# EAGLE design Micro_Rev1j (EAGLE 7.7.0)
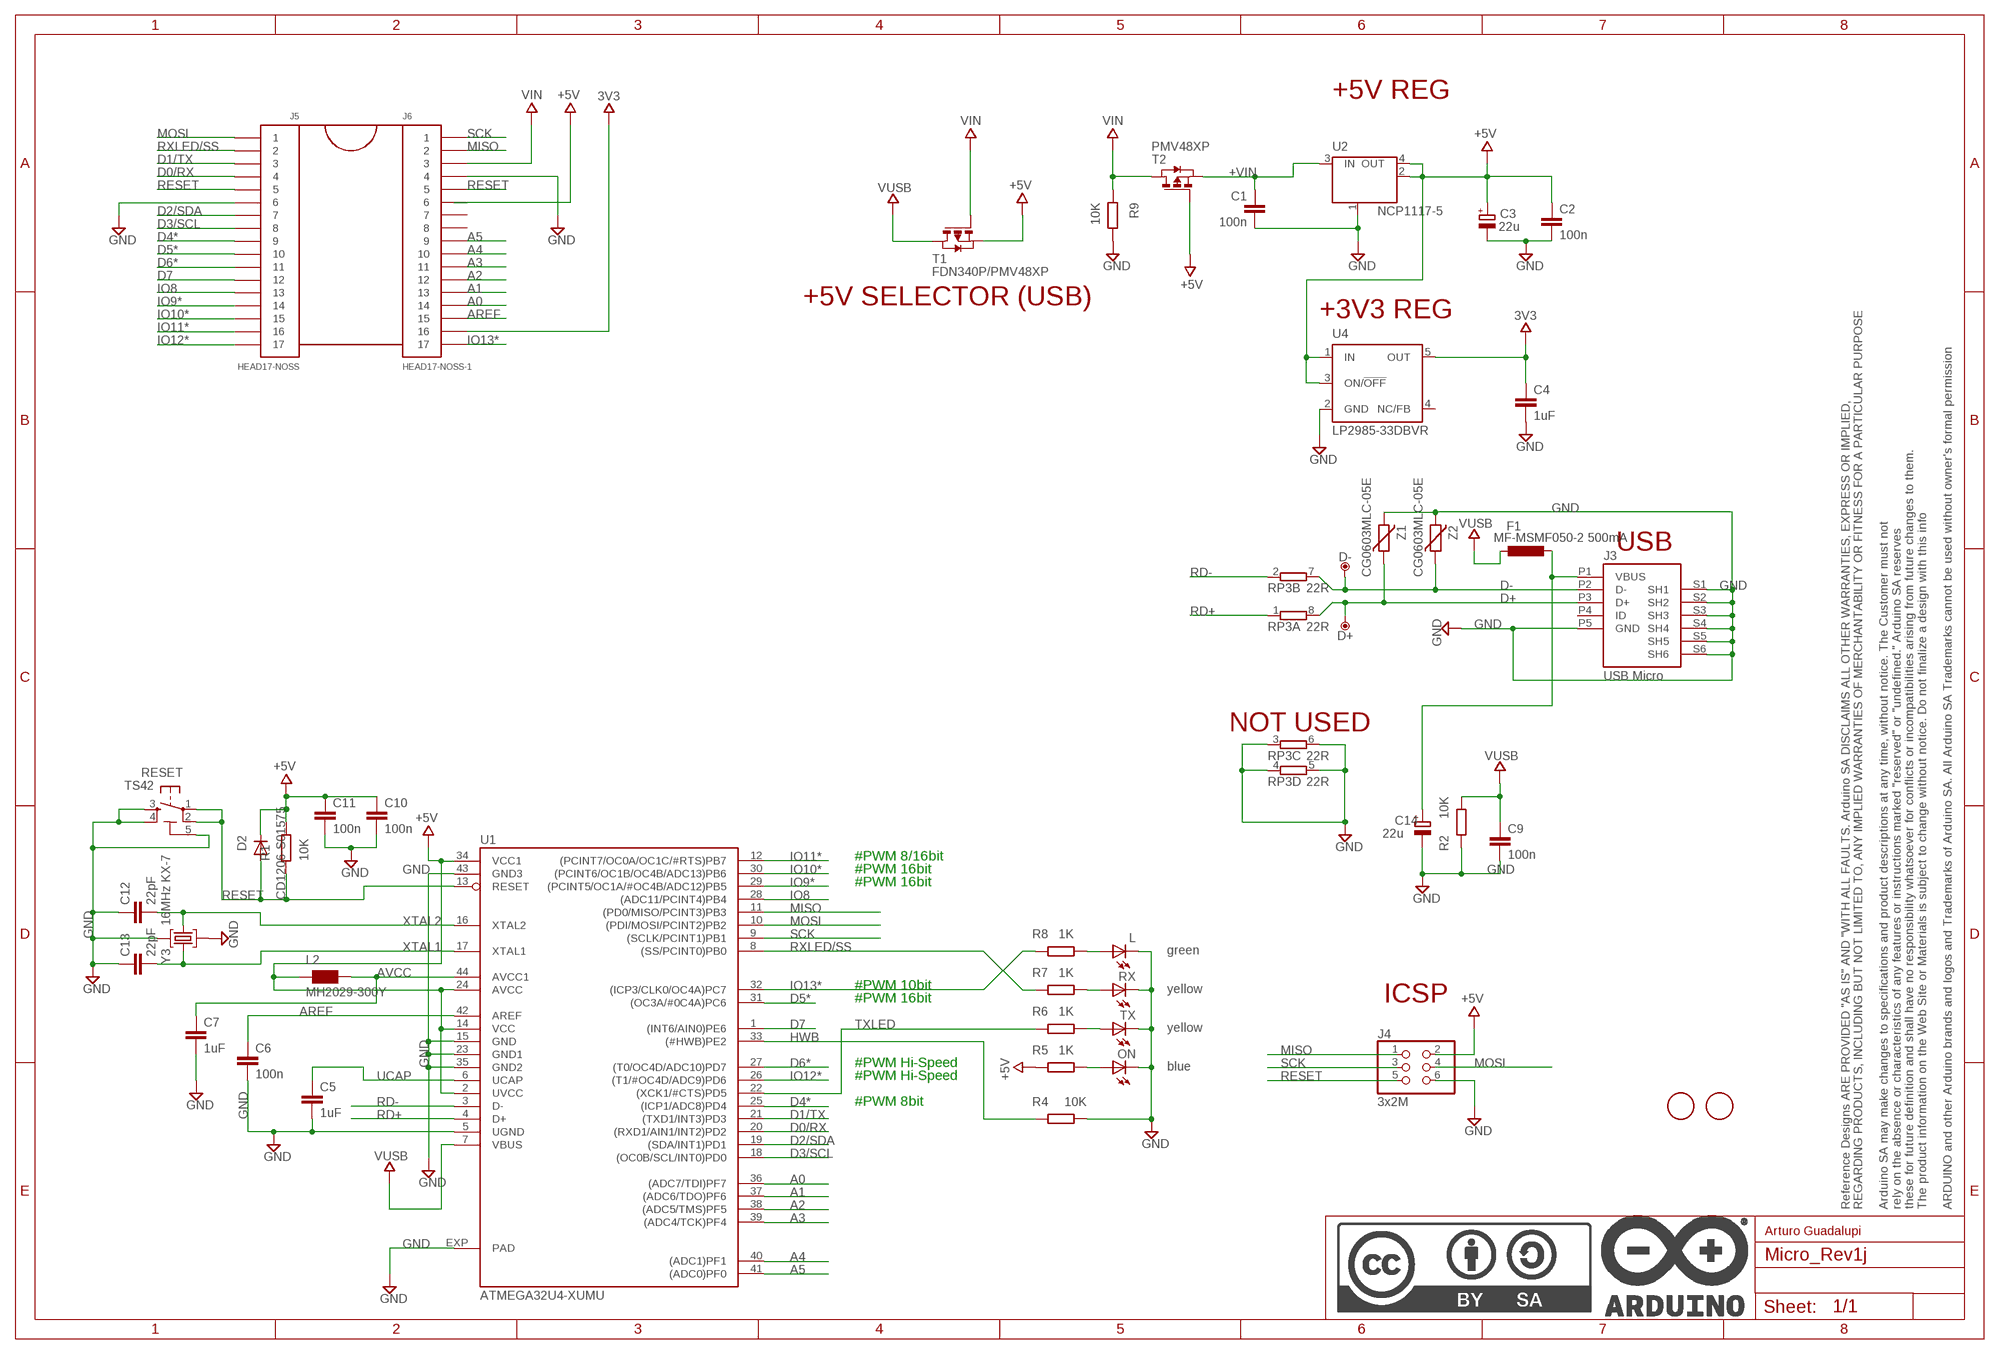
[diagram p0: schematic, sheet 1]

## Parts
C1  100n  C-EUC0402  [C0402]
C2  100n  C-EUC0402  [C0402]
C3  22u  CPOL-EUSMCB  [SMC_B]
C4  1uF  C-EUC0402  [C0402]
C5  1uF  C-EUC0402  [C0402]
C6  100n  C-EUC0402  [C0402]
C7  1uF  C-EUC0402  [C0402]
C9  100n  C-EUC0402  [C0402]
C10  100n  C-EUC0402  [C0402]
C11  100n  C-EUC0402  [C0402]
C12  22pF  C-EUC0402  [C0402]
C13  22pF  C-EUC0402  [C0402]
C14  22u  CPOL-EUSMCB  [SMC_B]
D2  CD1206-S01575  DIODE-MINIMELF  [MINIMELF]
D+  DNP  TPTP-1.00MM  [TP-1.00MM]
D-  DNP  TPTP-1.00MM  [TP-1.00MM]
F1  MF-MSMF050-2 500mA  L-EUL1812  [L1812]
FRAME1  DNP  A3-FRAME  [FRAME]
J3  USB Micro  USB-MICRO-LEGACY  [CON2_USB_MICRO_B_AT]
J4  3x2M  PINHD-2X3  [2X03]
J5  HEAD17-NOSS  [HEAD17-NOSS]
J6  HEAD17-NOSS-1  [HEAD17-NOSS-1]
L  green  LEDCHIPLED_0805  [CHIPLED_0805]
L2  MH2029-300Y  WE-CBF_0805  [0805]
ON  blue  LEDCHIPLED_0805  [CHIPLED_0805]
R1  10K  R-EU_R0402  [R0402]
R2  10K  R-EU_R0402  [R0402]
R4  10K  R-EU_R0402  [R0402]
R5  1K  R-EU_R0402  [R0402]
R6  1K  R-EU_R0402  [R0402]
R7  1K  R-EU_R0402  [R0402]
R8  1K  R-EU_R0402  [R0402]
R9  10K  R-EU_R0402  [R0402]
RESET  TS42  [TS42]
RP3  22R  4R-NCAY16  [CAY16]
RX  yellow  LEDCHIPLED_0805  [CHIPLED_0805]
T1  FDN340P/PMV48XP  PMOSSOT23  [SOT-23]
T2  PMV48XP  PMOSSOT23  [SOT-23]
TX  yellow  LEDCHIPLED_0805  [CHIPLED_0805]
U1  ATMEGA32U4-XUMU  [QFN44ML7X7]
U2  NCP1117-5  LINEAR_MC33269ST  [SOT223]
U4  LP2985-33DBVR  LP2985-XXDBVR33  [SOT23-DBV]
U$37  DNP  FIDUCIAL-1.5MM  [FD-1-1.5]
U$53  DNP  FIDUCIAL-1.5MM  [FD-1-1.5]
Y3  16MHz KX-7  CRYSTAL-3.2-2.5  [CRYSTAL-3.2-2.5]
Z1  CG0603MLC-05E  VARISTORCN0603  [CT/CN0603]
Z2  CG0603MLC-05E  VARISTORCN0603  [CT/CN0603]

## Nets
3V3: C4.1 J6.16 U4.5(OUT)
+5V: C2.1 C3.+ C10.1 C11.1 D2.C J4.2 J6.6 L2.1 R1.1 R5.1 T1.2(S) T2.3(G) U1.2(UVCC) U1.14(VCC) U1.24(AVCC) U1.34(VCC1) U2.2(OUT) U2.4(OUT) U4.1(IN) U4.3(ON/!OFF)
+VIN: C1.1 T2.2(S) U2.3(IN)
A0: J6.14 U1.36((ADC7/TDI)PF7)
A1: J6.13 U1.37((ADC6/TDO)PF6)
A2: J6.12 U1.38((ADC5/TMS)PF5)
A3: J6.11 U1.39((ADC4/TCK)PF4)
A4: J6.10 U1.40((ADC1)PF1)
A5: J6.9 U1.41((ADC0)PF0)
AREF: C6.1 J6.15 U1.42(AREF)
AVCC: C7.1 L2.2 U1.44(AVCC1)
D0/RX: J5.4 U1.20((RXD1/AIN1/INT2)PD2)
D1/TX: J5.3 U1.21((TXD1/INT3)PD3)
D2/SDA: J5.7 U1.19((SDA/INT1)PD1)
D3/SCL: J5.8 U1.18((OC0B/SCL/INT0)PD0)
D4*: J5.9 U1.25((ICP1/ADC8)PD4)
D5*: J5.10 U1.31((OC3A/#0C4A)PC6)
D6*: J5.11 U1.27((T0/OC4D/ADC10)PD7)
D7: J5.12 U1.1((INT6/AIN0)PE6)
D+: D+.X J3.P3(D+) RP3.8 Z1.1
D-: D-.X J3.P2(D-) RP3.7 Z2.1
GND: C1.2 C2.2 C3.- C4.2 C5.2 C6.2 C7.2 C9.2 C10.2 C11.2 C12.1 C13.1 C14.- J3.P5(GND) J3.S1(SH1) J3.S2(SH2) J3.S3(SH3) J3.S4(SH4) J3.S5(SH5) J3.S6(SH6) J4.6 J5.6 J6.4 L.C ON.C R2.1 R4.2 R9.1 RESET.3 RESET.4 RESET.5(5-GND) RP3.3 RP3.4 RP3.5 RP3.6 RX.C TX.C U1.5(UGND) U1.15(GND) U1.23(GND1) U1.35(GND2) U1.43(GND3) U1.EXP(PAD) U2.1(GND/ADJ) U4.2(GND) Y3.2(GND) Y3.4(GND) Z1.2 Z2.2
HWB: R4.1 U1.33((#HWB)PE2)
IO8: J5.13 U1.28((ADC11/PCINT4)PB4)
IO9*: J5.14 U1.29((PCINT5/OC1A/#OC4B/ADC12)PB5)
IO10*: J5.15 U1.30((PCINT6/OC1B/OC4B/ADC13)PB6)
IO11*: J5.16 U1.12((PCINT7/OC0A/OC1C/#RTS)PB7)
IO12*: J5.17 U1.26((T1/#OC4D/ADC9)PD6)
IO13*: J6.17 R8.1 U1.32((ICP3/CLK0/OC4A)PC7)
MISO: J4.1 J6.2 U1.11((PD0/MISO/PCINT3)PB3)
MOSI: J4.4 J5.1 U1.10((PDI/MOSI/PCINT2)PB2)
N$2: R7.2 RX.A
N$3: ON.A R5.2
N$4: R6.2 TX.A
N$7: L.A R8.2
RD+: RP3.1 U1.4(D+)
RD-: RP3.2 U1.3(D-)
RESET: D2.A J4.5 J5.5 J6.5 R1.2 RESET.1 RESET.2 U1.13(RESET)
RXLED/SS: J5.2 R7.1 U1.8((SS/PCINT0)PB0)
SCK: J4.3 J6.1 U1.9((SCLK/PCINT1)PB1)
TXLED: R6.1 U1.22((XCK1/#CTS)PD5)
UCAP: C5.1 U1.6(UCAP)
VIN: J6.3 R9.2 T1.3(G) T2.1(D)
VUSB: C9.1 F1.2 R2.2 T1.1(D) U1.7(VBUS)
VUSBD: C14.+ F1.1 J3.P1(VBUS)
XTAL1: C13.2 U1.17(XTAL1) Y3.3(C2)
XTAL2: C12.2 U1.16(XTAL2) Y3.1(C1)
Unconnected: J3.P4(ID) J6.7 J6.8 U4.4(NC/FB)

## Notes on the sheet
- +5V REG
- +5V SELECTOR (USB)
- +3V3 REG
- USB
- NOT USED
- #PWM 8/16bit
- #PWM 16bit
- #PWM 16bit
- #PWM 10bit
- #PWM 16bit | ICSP
- #PWM Hi-Speed
- #PWM Hi-Speed
- #PWM 8bit
- Arturo Guadalupi

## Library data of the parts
C1 C2 C4-C7 C9-C13 = gen_comp:C-EU: CAPACITOR, European symbol
C3 C14 = rcl:CPOL-EU: POLARIZED CAPACITOR, European symbol
D2 = diode:DIODE-: DIODE
D+ D- = Arduino-utility:TP: Testpoint; DATASHEET: DNP; DISTRIBUTOR-LINK: DNP; DISTRIBUTOR-PN: DNP; MANUFACTURER: DNP; MANUFACTURER-PN: DNP
F1 = rcl:L-EU: INDUCTOR, European symbol
FRAME1 = Arduino-utility:A3-FRAME; CODE-ARDUINO: DNP; DATASHEET: DNP; DISTRIBUTOR-LINK: DNP; DISTRIBUTOR-PN: DNP; MANUFACTURER: DNP; MANUFACTURER-PN: DNP; NOTE: DNP
J3 = Arduino-connectors:USB-MICRO-LEGACY; DATASHEET: http://media.digikey.com/pdf/Data%20Sheets/FCI%20PDFs/10118193-0001LF_Webpage.PDF; DISTRIBUTOR-LINK: http://www.digikey.it/product-detail/en/10118193-0001LF/609-4616-2-ND/2785388; DISTRIBUTOR-PN: 609-4616-2-ND; MANUFACTURER: FCI; MANUFACTURER-PN: 10118193-0001LF
J4 = gen_comp:PINHD-2X3: PIN HEADER
J5 = gen_comp:HEAD17-NOSS
J6 = gen_comp:HEAD17-NOSS-1
L ON RX TX = led:LED: LED
L2 = wuerth-elektronik:WE-CBF: SMD EMI Suppression Ferrite Beads
R1 R2 R4-R9 = gen_comp:R-EU_: RESISTOR, European symbol
RESET = Arduino:TS42: TS42 Dongnan Electronics Tact switch VDC 12V - 50mA
RP3 = resistor-dil:4R-N: Array Chip Resistor Source: RS Component / Phycomp
T1 T2 = zetex:PMOSSOT23: MOS FET
U1 = gen_comp:ATMEGA32U4-XU
U2 = gen_comp:LINEAR_MC33269ST*: Adjustable Output Low Dropout Voltage Regulator 800 mA Source: http://www.onsemi.com/pub/Collateral/MC33269-D.PDF
U4 = gen_comp:LP2985-XXDBVR: ULTRALOW-POWER 50-mA LOW-DROPOUT LINEAR REGULATORS 50-mA Low-Dropout Regulator Source: http://focus.ti.com/lit/ds/symlink/tps77001.pdf
U$37 U$53 = Arduino-utility:FIDUCIAL: Fiducial mount; DATASHEET: DNP; DISTRIBUTOR-LINK: DNP; DISTRIBUTOR-PN: DNP; MANUFACTURER: DNP; MANUFACTURER-PN: DNP
Y3 = gen_comp:CRYSTAL-3.2-2.5
Z1 Z2 = varistor:VARISTOR: VARISTOR

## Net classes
0 default: width 0.254 mm, drill 0.5 mm, clearance 0.203 mm

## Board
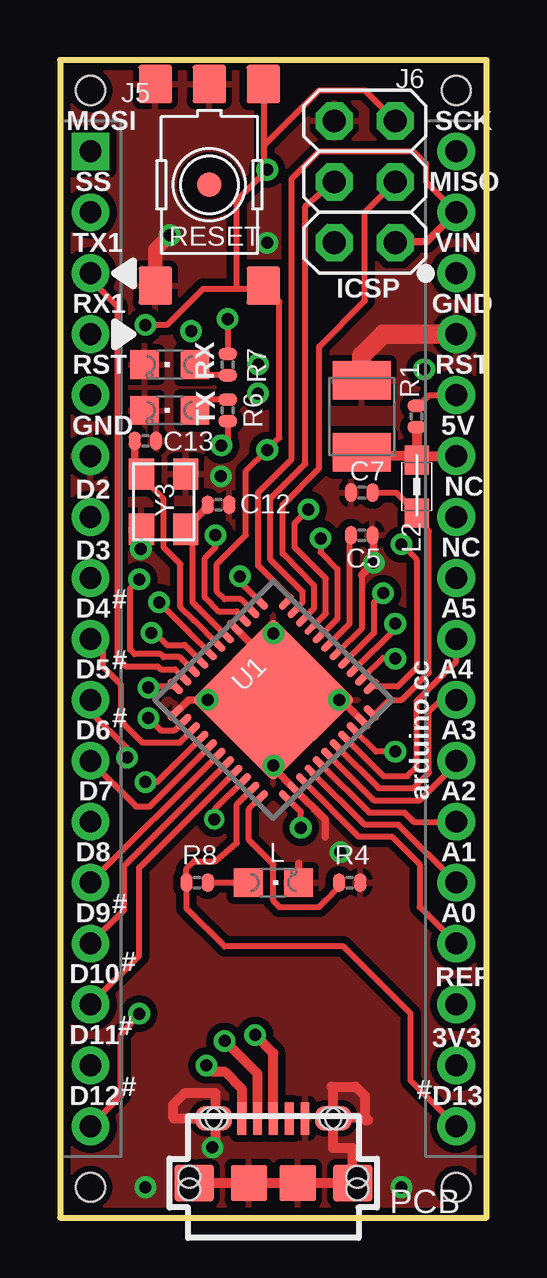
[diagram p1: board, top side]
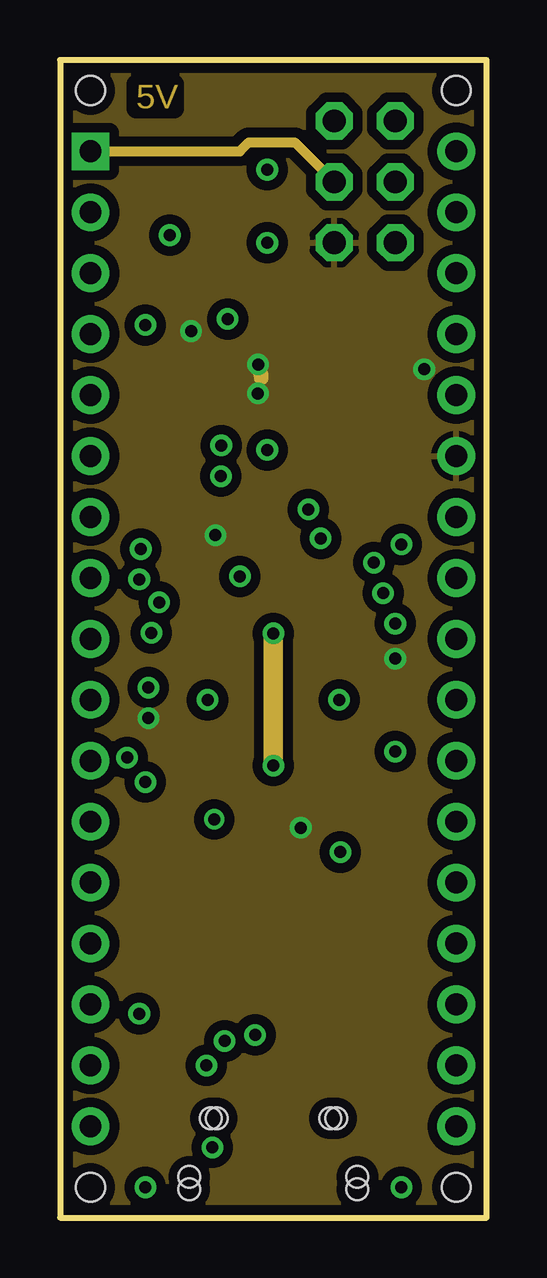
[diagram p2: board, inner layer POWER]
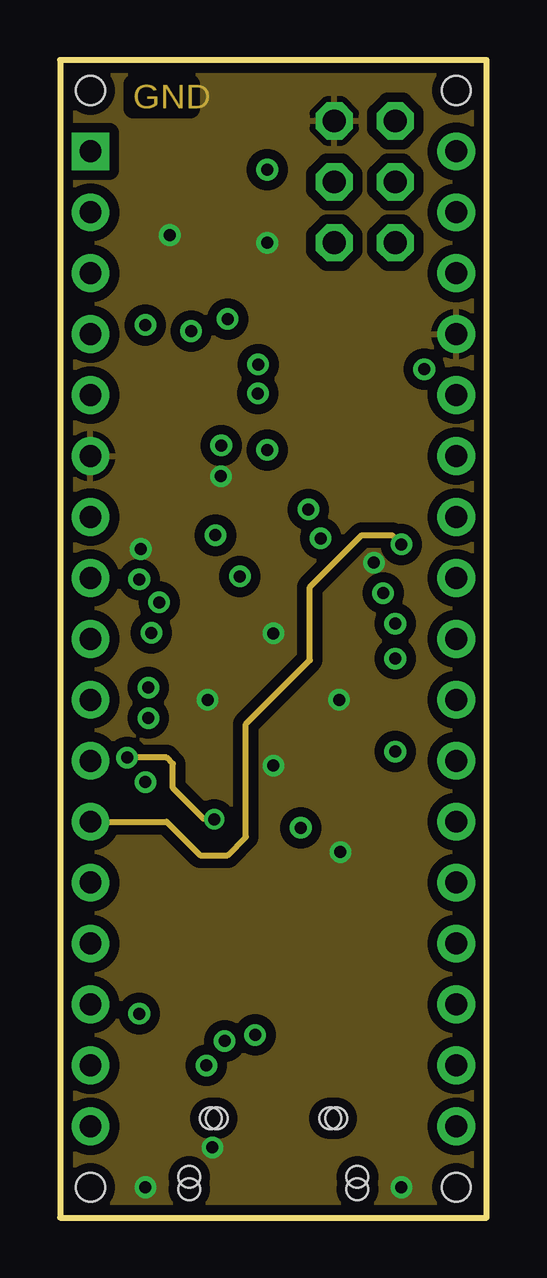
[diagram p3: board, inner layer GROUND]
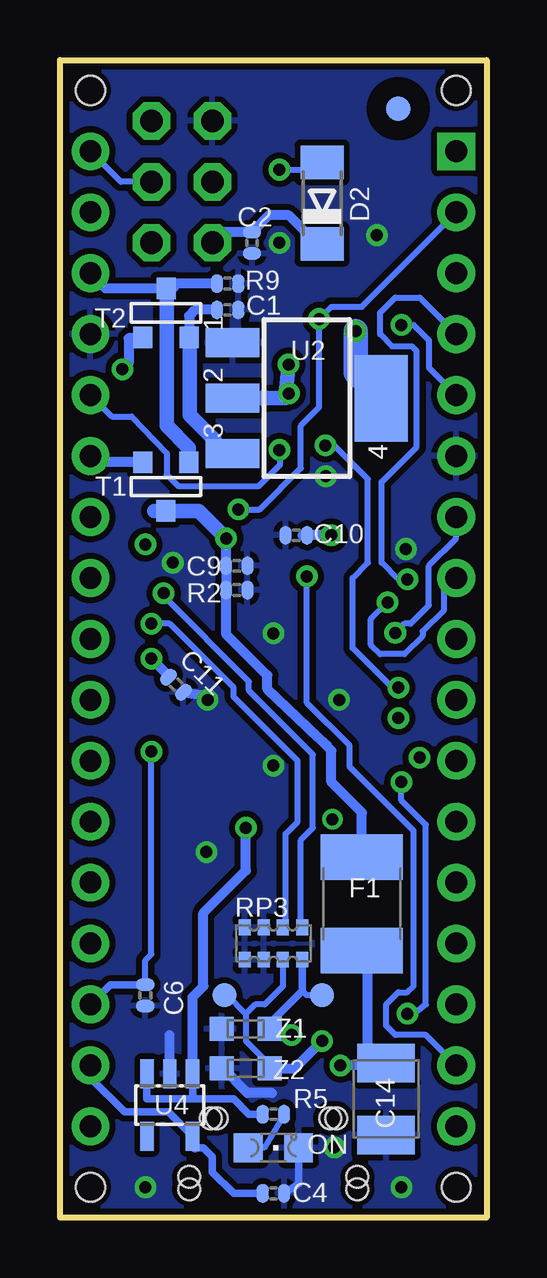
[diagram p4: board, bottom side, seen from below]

Size 17.78 x 48.26 mm. Coordinates in mm from the lower left corner, seen from the top.
Outline: 0,0 17.78,0 17.78,48.26 0,48.26 0,0
Copper layers (1*2*15*16): Top 0.035mm / dielectric 0.2mm / POWER 0.0175mm / dielectric 0.3mm / GROUND 0.0175mm / dielectric 0.2mm / Bottom 0.035mm
Design rules "SystemElettronica": minimum track width 6mil, minimum drill 0.499mm, track to track 6mil, track to pad 6mil, pad to pad 5mil, via to via 5mil, smd to smd 0mil, copper to edge 10mil, drill to drill 8mil, minimum pad ring 6mil, minimum via ring 4mil, stop-mask expansion 4mil, vias tented up to drill 25mil, thermal gap 10mil
Holes 1.2 mm at 1.27,1.27 16.51,1.27 1.27,46.99 16.51,46.99

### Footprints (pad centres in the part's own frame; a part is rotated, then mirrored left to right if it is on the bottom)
C0402 = smd 0.508 x 0.762: 1 -0.445,0; 2 0.445,0
SMC_B = smd 1.6 x 2.4: + -1.5,0; - 1.5,0
MINIMELF = smd 1.4 x 1.8: A 1.7,0; C -1.7,0
TP-1.00MM = smd 1 x 1 bottom: X 0,0
L1812 = smd 1.9 x 3.4: 1 -1.95,0; 2 1.95,0
CON2_USB_MICRO_B_AT = smd 0.406 x 1.346: P1 -1.321,2.692; P2 -0.66,2.692; P3 0,2.692; P4 0.66,2.692; P5 1.321,2.692 | smd 1.651 x 1.549: S1 -3.302,0; S2 3.302,0 | smd 1.524 x 1.016: S3 -2.489,2.692; S4 2.489,2.692 | smd 1.524 x 1.524: S5 -1.016,0; S6 1.016,0 | hole 0.9: -3.505,0.254; -3.505,-0.254; 3.505,0.254; 3.505,-0.254; -2.616,2.692; -2.362,2.692; 2.362,2.692; 2.616,2.692
2X03 = drill 0.95 pad 1.55 octagon: 1 -2.54,-1.27; 2 -2.54,1.27; 3 0,-1.27; 4 0,1.27; 5 2.54,-1.27; 6 2.54,1.27
HEAD17-NOSS = drill 0.914 pad 1.575 square: 1 0,0 | drill 0.914 pad 1.575: 2 2.54,0; 3 5.08,0; 4 7.62,0; 5 10.16,0; 6 12.7,0; 7 15.24,0; 8 17.78,0; 9 20.32,0; 10 22.86,0; 11 25.4,0; 12 27.94,0; 13 30.48,0; 14 33.02,0; 15 35.56,0; 16 38.1,0; 17 40.64,0
HEAD17-NOSS-1 = drill 0.914 pad 1.575: 1 0,0; 2 2.54,0; 3 5.08,0; 4 7.62,0; 5 10.16,0; 6 12.7,0; 7 15.24,0; 8 17.78,0; 9 20.32,0; 10 22.86,0; 11 25.4,0; 12 27.94,0; 13 30.48,0; 14 33.02,0; 15 35.56,0; 16 38.1,0; 17 40.64,0
CHIPLED_0805 = smd 1.2 x 1.2: A 0,-1.05; C 0,1.05
0805 = smd 1.2 x 1: 1 -1.1,0; 2 1.1,0
R0402 = smd 0.508 x 0.762: 1 -0.445,0; 2 0.445,0
TS42 = smd 1.6 x 1.4: 1 -4.2,2.25; 2 4.2,2.25; 3 -4.2,-2.25; 4 4.2,-2.25; 5 -4.2,0
CAY16 = smd 0.5 x 0.65: 1 -1.2,-0.675; 2 -0.4,-0.675; 3 0.4,-0.675; 4 1.2,-0.675; 5 1.2,0.675; 6 0.4,0.675; 7 -0.4,0.675; 8 -1.2,0.675
SOT-23 = smd 0.787 x 0.889: 1 0.025,-1.016; 2 -0.94,1.016; 3 0.991,1.016
QFN44ML7X7 = smd 0.75 x 0.275: 1 -3.275,2.5; 2 -3.275,2; 3 -3.275,1.5; 4 -3.275,1; 5 -3.275,0.5; 6 -3.275,0; 7 -3.275,-0.5; 8 -3.275,-1; 9 -3.275,-1.5; 10 -3.275,-2; 11 -3.275,-2.5; 23 3.275,-2.5; 24 3.275,-2; 25 3.275,-1.5; 26 3.275,-1; 27 3.275,-0.5; 28 3.275,0; 29 3.275,0.5; 30 3.275,1; 31 3.275,1.5; 32 3.275,2; 33 3.275,2.5 | smd 0.275 x 0.75: 12 -2.5,-3.275; 13 -2,-3.275; 14 -1.5,-3.275; 15 -1,-3.275; 16 -0.5,-3.275; 17 0,-3.275; 18 0.5,-3.275; 19 1,-3.275; 20 1.5,-3.275; 21 2,-3.275; 22 2.5,-3.275; 34 2.5,3.275; 35 2,3.275; 36 1.5,3.275; 37 1,3.275; 38 0.5,3.275; 39 0,3.275; 40 -0.5,3.275; 41 -1,3.275; 42 -1.5,3.275; 43 -2,3.275; 44 -2.5,3.275 | smd 4.826 x 4.826: EXP 0,0
SOT223 = smd 1.219 x 2.235: 1 -2.311,-3.099; 2 0,-3.099; 3 2.311,-3.099 | smd 3.6 x 2.2: 4 0,3.099
SOT23-DBV = smd 0.55 x 1.2: 1 -0.95,-1.3; 2 0,-1.3; 3 0.95,-1.3; 4 0.95,1.3; 5 -0.95,1.3
FD-1-1.5 = smd 1.016 x 1.016: P$1 0,0
CRYSTAL-3.2-2.5 = smd 1.3 x 1.05: 1 -1.15,-0.925; 2 1.15,-0.925; 3 1.15,0.925; 4 -1.15,0.925
CT/CN0603 = smd 1 x 1: 1 -1,0; 2 1,0

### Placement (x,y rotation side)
C1  10.79,37.85 0 bottom
C2  9.78,40.64 270 bottom
C3  12.57,33.4 90 top
C4  8.89,1.02 0 bottom
C5  12.57,28.45 0 top
C6  14.22,9.27 270 bottom
C7  12.57,30.23 180 top
C9  10.41,27.18 0 bottom
C10  7.94,28.45 180 bottom
C11  12.95,22.23 315 bottom
C12  6.6,29.72 180 top
C13  3.56,32.38 180 top
C14  4.19,4.95 270 bottom
D2  6.86,42.29 90 bottom
D+  6.86,9.27 0 top
D-  10.92,9.27 0 top
F1  5.21,13.08 90 bottom
FRAME1  0,0 0 top
J3  8.89,1.45 0 top
J4  12.7,43.18 90 top
J5  1.27,44.45 270 top
J6  16.51,44.45 270 top
L  8.89,13.97 270 top
L2  14.86,30.48 270 top
ON  8.89,2.92 270 bottom
R1  14.86,33.4 90 top
R2  10.41,26.16 180 bottom
R4  12.06,13.97 0 top
R5  8.89,4.32 0 bottom
R6  6.99,33.66 90 top
R7  6.99,35.56 270 top
R8  5.71,13.97 0 top
R9  10.79,38.94 180 bottom
RESET  6.22,43.05 270 top
RP3  8.89,11.43 180 bottom
RX  4.57,35.56 90 top
T1  13.4,30.48 0 bottom
T2  13.34,37.72 180 bottom
TX  4.57,33.66 90 top
U1  8.89,21.59 225 top
U2  7.49,34.16 270 bottom
U4  13.21,4.7 180 bottom
U$37  6.22,43.05 0 top
U$53  3.68,46.23 0 bottom
Y3  4.32,29.84 90 top
Z1  10.03,7.87 180 bottom
Z2  10.03,6.22 180 bottom

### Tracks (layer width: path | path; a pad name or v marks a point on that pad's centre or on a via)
3V3
  Bottom 0.305: U4.5 13.28,4.42 15.09,4.42 16.51,5.84 J6.16 | 12.16,2.92 11.81,2.92 11.43,2.54 11.43,1.91 10.54,1.02 C4.1
  Bottom 0.406: 12.16,2.92 U4.5
+5V  (via drill 0.5 pad 0.9)
  Top 0.254: U1.24 4.79,20.32 4.19,20.32 v3.68,20.83 | U1.14 7.37,25.27 6.6,25.27 6.03,25.84 6.03,27.5 6.48,27.94 v6.48,28.45 | U1.2 13.46,23.33 v13.97,23.3 | U1.34 10.03,16.91 v10.03,16.26
  Top 0.406: R1.1 L2.1 14.73,31.58 14.73,31.75 | 14.73,31.75 J6.6 | 14.73,31.75 12.57,31.75 C3.+
  POWER 0.61: v8.26,35.57 8.38,35.06 8.38,35.14 8.39,35.14 8.39,35
  Bottom 0.305: U4.1 12.26,4.95 | 12.26,4.95 10.54,4.95 9.91,4.32 R5.1 | U4.3 14.16,4.95 12.26,4.95
  Bottom 0.406: v10.03,16.26 10.03,14.48 11.81,12.7 11.81,9.65 12.26,9.21 U4.1 | C11.1 13.41,22.75 v13.97,23.3 | 7.68,28.45 C10.1 v6.48,28.45 | D2.C 7.06,40.59 8.26,41.78 9.08,41.78 C2.1 10.99,41.08 J4.2 | T1.2 16.26,31.5 J6.6 | T2.3 14.92,36.66 14.92,35.62 v15.18,35.37
  Bottom 0.61: U2.2 8.38,34.16 v8.26,35.57
  Bottom 1.016: v5.46,36.96 5.46,35.23 U2.4
  other vias: 8.25,34.36
  pour POWER (isolate 0.406): -0.64,48.9 18.41,48.9 18.41,-0.64 -0.64,-0.64
+VIN
  Bottom 0.406: C1.1 12.14,37.85 12.39,37.59 T2.2
  Bottom 0.61: U2.3 11.34,31.85 11.34,32.42 12.38,33.47 12.38,35.99 T2.2
A0
  Top 0.254: U1.36 12.45,15.88 13.84,15.88 14.99,14.73 14.99,12.95 J6.14
A1
  Top 0.254: U1.37 12.7,16.38 14.1,16.38 J6.13
A2
  Top 0.254: U1.38 12.88,16.89 | 12.88,16.89 | 12.88,16.89 14.35,16.89 14.73,16.51 J6.12
A3
  Top 0.254: U1.39 13.08,17.4 14.99,17.4 16.26,18.67 J6.11
A4
  Top 0.254: U1.40 13.28,17.91 14.73,17.91 15.37,18.54 15.37,21.08 15.88,21.59 J6.10
A5
  Top 0.254: U1.41 13.48,18.41 14.48,18.41 14.86,18.8 14.86,21.54 16.51,23.19 J6.9
AREF  (via drill 0.5 pad 0.9)
  Top 0.254: U1.42 13.17,19.43 v13.97,19.43
  Bottom 0.254: v13.97,19.43 13.97,10.99 14.22,10.73 C6.1
  Bottom 0.305: C6.1 15.68,9.72 J6.15
AVCC
  Top 0.254: U1.44 13.17,21.04 13.72,21.59 14.24,21.59 15.37,22.72 15.37,28.62 L2.2 14.01,30.23 C7.1
D0/RX  (via drill 0.5 pad 0.9)
  Top 0.254: U1.20 4.99,23.37 4.32,23.37 4.19,23.5 3.11,23.5 2.92,23.69 2.92,26.23 v3.3,26.61
  Bottom 0.254: v3.3,26.61 3.68,26.61 4.38,27.3 4.38,30.67 2.92,32.13 2.92,36.13 3.11,36.32 3.94,36.32 4.45,36.83 4.45,37.72 3.81,38.35 2.79,38.35 J5.4
D1/TX
  Top 0.254: U1.21 4.79,22.86 4.19,22.86 4.06,22.99 2.73,22.99 2.41,23.3 2.41,37.97 1.27,39.12 J5.3
D2/SDA  (via drill 0.5 pad 0.9)
  Top 0.254: U1.19 5.19,23.88 4.45,23.88 3.94,24.38 v3.81,24.38
  Bottom 0.254: v3.81,24.38 3.43,24.77 3.17,24.77 2.41,25.53 2.41,27.18 1.27,28.32 J5.7
D3/SCL  (via drill 0.5 pad 0.9)
  Top 0.254: U1.18 5.39,24.38 5.4,24.38 v4.13,25.65
  Bottom 0.254: v4.13,25.65 4.83,24.96 4.83,23.88 4.45,23.5 3.43,23.5 2.67,24.26 2.67,24.45 1.78,25.34 1.78,26.16 J5.8
D4*
  Top 0.254: U1.25 4.99,19.81 3.43,19.81 2.54,20.7 2.54,22.23 1.78,22.99 1.78,23.62 J5.9
D5*  (via drill 0.5 pad 0.85, 0.5 pad 0.9)
  Top 0.254: U1.31 6.48,17.06 v6.43,16.61 | J5.10 1.27,21.08 2.79,19.56 v2.79,19.18
  GROUND 0.254: v2.79,19.18 4.45,19.18 4.7,18.92 4.7,17.91 5.97,16.64 v6.43,16.61
D6*
  Top 0.254: U1.27 3.74,17.14 3.17,17.14 J5.11
D7  (via drill 0.5 pad 0.9)
  Top 0.254: U1.1 14.06,22.14 14.06,22.13 14.86,22.94 14.86,27.43 v14.22,28.07
  GROUND 0.254: J5.12 4.45,16.51 5.84,15.11 6.99,15.11 7.75,15.88 7.75,20.57 10.41,23.24 10.41,26.29 12.57,28.45 13.84,28.45 v14.22,28.07
D+  (via drill 0.5 pad 0.9)
  Top 0.406: J3.P3 8.89,6.86 v8.13,7.62
  Bottom 0.254: D+.X 7.51,9.27 7.69,9.46
  Bottom 0.305: RP3.8 7.69,9.46 9.27,7.87 9.14,7.87
  Bottom 0.406: v8.13,7.62 Z1.1 9.14,7.87
D-  (via drill 0.5 pad 0.9)
  Top 0.406: J3.P2 8.23,5.99 v6.86,7.37
  Bottom 0.254: RP3.7 8.49,9.65 9.25,8.89 9.65,8.89 10.03,8.51 | 10.03,8.51 10.03,7.37 9.03,6.37 Z2.1 | D-.X 10.79,9.27 10.03,8.51
  Bottom 0.406: Z2.1 8,6.22 v6.86,7.37
GND  (via drill 0.5 pad 0.9)
  Top 0.254: U1.EXP v8.89,24.36 | U1.5 12.57,24.57 12.57,26.8 | 13.04,28.19 C5.2
  Top 0.305: U1.EXP 8.89,18.76 U1.35 11.05,16.6 11.05,15.88 | U1.23 5.35,21.59 U1.EXP | U1.15 8.89,23 U1.EXP | L.C 9.94,14.77 | 12.57,26.8 v13.08,27.3 13.08,28.28 13.04,28.19 | U1.43 11.72,21.59 v11.63,21.59
  Top 0.406: J3.S1 J3.S2 12.19,2.9 11.38,2.9 J3.S4 | 6.22,3.05 v6.35,2.93 6.48,3.05 6.48,5.21 5.21,5.21 4.7,4.7 4.7,4.19 4.75,4.14 J3.S3 | J3.S4 11.38,5.38 11.3,5.46 12.32,5.46 12.7,5.08 12.7,4.19 12.83,4.06 12.7,4.06 12.57,4.19 11.43,4.19 J3.S4
  Top 0.61: RESET.4 3.97,40.36 v4.57,40.96 | Y3.4 3.39,28.09 v3.37,27.88
  Top 0.813: C3.- 12.57,35.94 13.46,36.83 J6.4
  POWER 0.813: v8.89,24.36 v8.89,18.85
  Bottom 0.305: ON.C 7.84,1.42 C4.2
  Bottom 0.406: U4.2 13.21,7.62 | C11.2 11.81,21.77 v11.63,21.59 | 8.95,5.21 9.97,5.21 11.05,6.29
  other vias: 11.68,15.24 6.71,30.91 6.15,21.59 3.56,1.27 14.22,1.27 8.64,40.64
  pour GROUND (isolate 0.406): -1.27,49.53 19.05,49.53 19.05,-1.27 -1.27,-1.27
  pour Bottom (isolate 0.254): 19.68,50.16 -1.91,50.16 -1.91,-1.91 19.68,-1.91
  pour Top (isolate 0.305): -2.54,50.8 20.32,50.8 20.32,-2.54 -2.54,-2.54
HWB
  Top 0.254: U1.33 7.87,17.04 7.87,15.75 8.89,14.73 8.89,13.21 9.14,12.95 10.79,12.95 11.05,13.21 11.56,13.73 R4.1
IO8
  Top 0.254: J5.13 U1.28
IO9*
  Top 0.254: U1.29 2.67,14.66 2.67,12.83 J5.14
IO10*
  Top 0.254: U1.30 3.3,14.59 3.3,10.92 J5.15
IO11*  (via drill 0.5 pad 0.9)
  Top 0.254: U1.12 7.49,26.52 v7.49,26.73
  Bottom 0.254: v7.49,26.73 7.49,21.46 5.71,19.68 5.71,18.8 3.05,16.13 3.05,9.65 3.3,9.4 3.68,9.4 4.19,8.89 4.19,8 3.81,7.62 2.54,7.62 J5.16
IO12*  (via drill 0.5 pad 0.9)
  Top 0.254: J5.17 2.54,5.08 2.54,7.62 v3.3,8.51 | U1.26 4.05,18.16 v3.56,18.16
  Bottom 0.254: v3.3,8.51 3.05,8.51 2.54,8.89 2.54,16.38 3.56,17.4 v3.56,18.16
IO13*
  Top 0.254: J6.17 14.61,5.71 14.61,8.51 11.81,11.3 6.86,11.3 5.27,12.89 R8.1 5.27,14.54 5.59,14.86 6.48,14.86 7.37,15.62 7.37,17.24 U1.32
MISO
  Top 0.254: U1.11 9.53,25.76 9.53,25.91 8.26,27.18 8.26,30.23 9.65,31.62 9.65,43.31 10.79,44.45 14.73,44.45 15.24,43.94 15.24,43.18 J6.2
  Top 0.305: J6.2 15.28,40.68 14.01,40.68 J4.1
MOSI
  Top 0.254: U1.10 10.11,25.66 10.11,26.09 8.76,27.43 8.76,29.97 10.22,31.43 10.22,42.16 J4.4
  POWER 0.406: J5.1 7.49,44.45 7.87,44.83 9.78,44.83 J4.4
N$2
  Top 0.254: R7.2 5.91,35.12 5.46,35.56 RX.A 5.59,35.56
N$3
  Bottom 0.254: R5.2 9.27,2.92 ON.A
N$4
  Top 0.254: R6.2 6.07,34.1 TX.A
N$7
  Top 0.254: R8.2 L.A
RD+  (via drill 0.5 pad 0.9)
  Top 0.254: U1.4 13.08,24.37 13.08,25.65 v13.46,26.04
  Bottom 0.254: v13.46,26.04 13.46,25.91 9.91,22.35 9.91,21.97 7.24,19.3 7.24,16.26 7.75,15.75 7.75,11.91 RP3.1
RD-  (via drill 0.5 pad 0.9)
  Top 0.254: U1.3 13.97,24.55 v13.97,24.77
  Bottom 0.254: v13.97,24.77 13.21,24.77 10.54,22.1 10.54,21.72 7.87,19.05 7.87,16.51 8.38,16 8.38,11.96 RP3.2
RESET  (via drill 0.5 pad 0.9)
  Top 0.254: U1.13 7.53,25.78 6.86,25.78 6.54,26.1 6.54,27.24 7.75,28.45 7.75,31.11 v8.64,32 9.14,32.51 9.14,38.18 RESET.2 | v8.64,43.69 8.51,43.69 8.51,43.81 | 8.51,43.81 8.51,44.7 | 8.51,44.7 10.79,46.99 12.7,46.99 J4.5 | v3.56,37.21 4.45,37.21 5.96,38.73 8.51,38.73 8.38,38.85 8.38,38.86 8.51,38.86 | RESET.2 8.64,38.85 8.64,38.73 8.51,38.73 | 8.51,38.82 RESET.2 | 8.22,39.11 RESET.2 | RESET.2 8.45,38.83 8.45,38.92 8.47,38.77 | v8.64,43.69 7.37,42.42 7.37,38.73 8.51,38.73 | 8.51,38.73 8.51,38.86 | 8.51,38.86 8.47,38.9 RESET.2 | 8.47,38.77 RESET.2 | 8.47,38.77 8.51,38.73 | 14.9,33.85 14.95,33.85 15.39,34.29 J6.5 | v8.64,43.69 8.51,43.81 | 8.51,44.7 8.51,47.22 RESET.1
  Top 0.305: 14.9,33.85 R1.2
  Bottom 0.254: J5.5 2.41,35.43 2.41,36.58 3.05,37.21 v3.56,37.21 | J6.5 15.62,33.4 14.8,33.4 13.34,31.88 13.34,30.99 12.83,30.48 9.53,30.48 8.61,31.39 8.61,31.85 v8.64,32 | v8.64,43.69 6.86,43.69 D2.A 6.86,44.07
RXLED/SS  (via drill 0.5 pad 0.9)
  Top 0.254: U1.8 11.07,25.19 11.07,26.64 9.78,27.94 9.78,28.96 v10.35,29.53 | v6.99,37.47 R7.1
  Bottom 0.254: v10.35,29.53 9.46,29.53 7.75,31.24 7.75,33.02 6.99,33.78 v6.99,37.47 6.48,37.97 5.21,37.97 J5.2
SCK
  Top 0.254: U1.9 10.59,25.41 10.59,26.34 9.27,27.69 9.27,29.72 10.79,31.24 10.79,36.32 12.7,38.23 12.7,41.91 J4.3
  Bottom 0.254: J4.3 15.24,43.18 J6.1
TXLED  (via drill 0.5 pad 0.9)
  Top 0.254: U1.22 3.77,22.14 v3.68,22.1 | R6.1 6.99,32.46 v6.72,32.19
  Bottom 0.254: v3.68,22.1 3.94,22.1 5.59,23.75 5.59,26.67 4.95,27.3 4.95,30.79 6.36,32.19 v6.72,32.19
UCAP
  Top 0.254: U1.6 12.06,24.77 12.06,28.45 12.08,28.43 C5.1
VIN
  Bottom 0.406: J6.3 15.88,38.73 T2.1 13.08,38.73 12.9,38.94 R9.2
  Bottom 0.61: T1.3 12.41,32.09 13.34,33.02 13.34,38.2 T2.1
VUSB  (via drill 0.5 pad 0.9)
  Top 0.254: U1.7 11.56,24.96 11.56,27.05 10.86,27.75 v10.86,28.32
  Bottom 0.254: 13.72,29.46 13.84,29.46
  Bottom 0.406: 6.6,19.62 6.83,19.84 7.03,20.03 | 7.03,20.03 9.14,22.04 9.14,22.61 10.83,24.3 10.86,24.36 R2.2 C9.1 v10.86,28.32 10.82,28.42 10.9,28.42 | F1.2 5.21,16.89 6.48,18.16 6.48,19.47 7.03,20.03
  Bottom 0.61: 13.84,29.46 T1.1 | T1.1 13.72,29.46 | T1.1 12,29.46 v10.86,28.32
VUSBD  (via drill 0.5 pad 0.9)
  Top 0.406: J3.P1 7.57,5.38 6.86,6.1 6.35,6.1 v6.1,6.35
  Bottom 0.406: F1.1 4.95,10.62 4.95,7.21 C14.+ 4.09,6.35 v6.1,6.35
XTAL1
  Top 0.254: U1.17 5.59,24.89 5.02,25.46 5.02,27.24 4.32,27.94 4.32,29.97 3.46,30.83 | 3.56,30.83 3.46,30.83 | 3.46,30.83 3.43,30.86
  Top 0.305: C13.2 3.11,30.97 Y3.3 3.56,30.83
XTAL2
  Top 0.254: U1.16 5.79,25.4 5.52,25.65 5.52,25.72 5.52,28.37 5.23,28.68 Y3.1 5.21,28.7
  Top 0.305: C12.2 6.16,29.65 5.59,29.08 5.59,29.04 Y3.1

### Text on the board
POWER: 5V
GROUND: GND
tPlace: MOSI | SCK | SS | MISO | TX1 | VIN | RX1 | ICSP | GND | RST | RX | RST | GND | TX | 5V | D2 | NC | NC | D3 | D4 | # | A5 | # | D5 | A4 | D6 | # | A3 | D7 | A2 | D8 | A1 | # | D9 | A0 | D10 | # | REF | # | D11 | 3V3 | D12 | # | # | D13
tNames: arduino.cc
test-probe: MICRO / TEST POINTS | ISP1_4 | ISP1_3 | SS | ISP1_1 | 0 | DC_VIN+ | 1 | 5V_REF | DC_VIN- | ISP1_5 | USB1_GND | USB1_5V | 2 | 3 | 4 | A5 | 5 | A4 | 6 | A3 | 7 | A2 | 8 | A1 | 9 | A0 | USB_D+ | USB_D- | 10 | AREF | 11 | 3V3 | 12 | 13

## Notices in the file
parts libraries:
Arduino-utility: Copyright (c) 2016-2017 Arduino LLC. All right reserved.
